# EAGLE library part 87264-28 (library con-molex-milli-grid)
RECEPTACAL
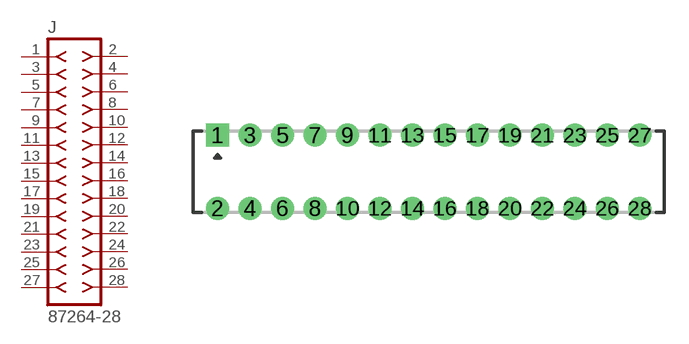
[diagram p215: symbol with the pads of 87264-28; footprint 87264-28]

Designator prefix J

## 87264-28  [87264-28]
1  1  pas
2  2  pas
3  3  pas
4  4  pas
5  5  pas
6  6  pas
7  7  pas
8  8  pas
9  9  pas
10  10  pas
11  11  pas
12  12  pas
13  13  pas
14  14  pas
15  15  pas
16  16  pas
17  17  pas
18  18  pas
19  19  pas
20  20  pas
21  21  pas
22  22  pas
23  23  pas
24  24  pas
25  25  pas
26  26  pas
27  27  pas
28  28  pas

## Footprint 87264-28 (pad centres in mm)
RECEPTACAL Dual Row, Side Entry
drill 0.914 square: 1 -13,2.25
drill 0.914: 2 -13,-2.25; 3 -11,2.25; 4 -11,-2.25; 5 -9,2.25; 6 -9,-2.25; 7 -7,2.25; 8 -7,-2.25; 9 -5,2.25; 10 -5,-2.25; 11 -3,2.25; 12 -3,-2.25; 13 -1,2.25; 14 -1,-2.25; 15 1,2.25; 16 1,-2.25; 17 3,2.25; 18 3,-2.25; 19 5,2.25; 20 5,-2.25; 21 7,2.25; 22 7,-2.25; 23 9,2.25; 24 9,-2.25; 25 11,2.25; 26 11,-2.25; 27 13,2.25; 28 13,-2.25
